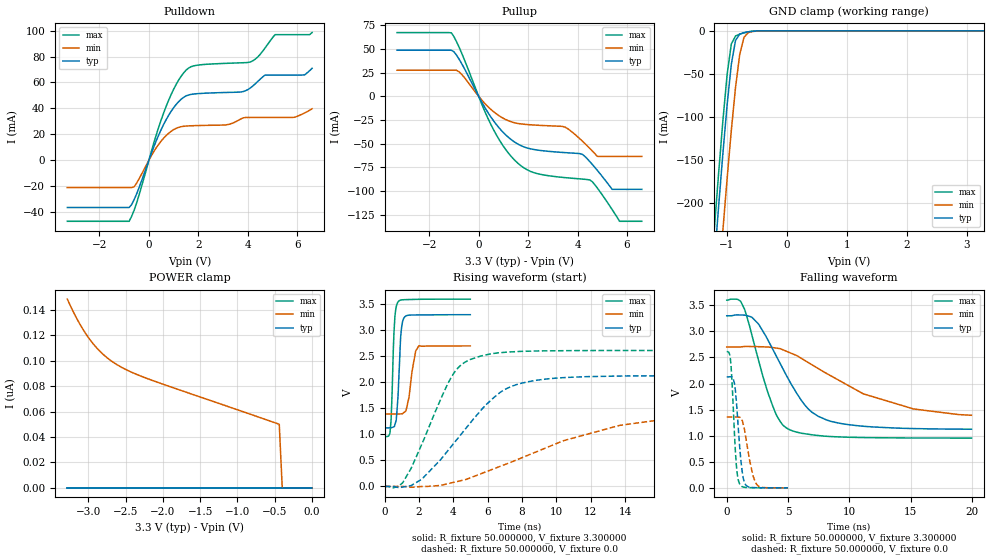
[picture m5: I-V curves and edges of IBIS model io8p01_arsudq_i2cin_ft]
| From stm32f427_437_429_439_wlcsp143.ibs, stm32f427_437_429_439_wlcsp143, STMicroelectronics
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|   Model io8p01_arsudq_i2cin_ft
[Model]  io8p01_arsudq_i2cin_ft
Model_type I/O
Polarity   Non-Inverting
Enable   Active-Low
Vinl =   0.990000V
Vinh =   2.310000V
Vmeas =  1.650000V
Cref =   50.000000pF
Rref =   100.000000M
Vref =   0.0V
C_comp   2.280000pF   2.217100pF   2.355700pF
[Temperature Range]   25.000000   0.125000k   -40.000000
[Pullup Reference]   3.300000V   2.700000V   3.600000V
[Pulldown Reference]   0.0V   0.0V   0.0V
[POWER Clamp Reference]   3.300000V   2.700000V   3.600000V
[GND Clamp Reference]   0.0V   0.0V   0.0V
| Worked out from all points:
|   slope of the pulldown table from 0 to 0.495 V, typ, clamps not added: 20.9 ohm
|   slope of the pullup table from 0 to 0.495 V, typ, clamps not added: 22.6 ohm
|   GND clamp passes 1 mA (typ) near -0.62 V on its own axis
|   rising waveform, R_fixture 50.000000, V_fixture 3.300000: 20-80 % time 192ps typ, 341ps min, 165ps max; typ from 1.12 V to 3.3 V
|   rising waveform, R_fixture 50.000000, V_fixture 0.0: 20-80 % time 3.34ns typ, 6.91ns min, 2.09ns max; typ from 0 V to 2.13 V
|   falling waveform, R_fixture 50.000000, V_fixture 3.300000: 20-80 % time 3.18ns typ, 6.84ns min, 2ns max; typ from 3.3 V to 1.12 V
|   falling waveform, R_fixture 50.000000, V_fixture 0.0: 20-80 % time 434ps typ, 633ps min, 342ps max; typ from 2.13 V to 0 V
[Pulldown]
|Voltage   I(typ)   I(min)   I(max)
-3.3V     -36.46mA   -21.09mA   -47.09mA
-800mV    -36.46mA   -21.09mA   -47.09mA
-600mV    -30.5mA    -20.54mA   -38.69mA
700mV     31.4mA     19.11mA    41.71mA
1.2V      45.15mA    25.37mA    61.75mA
1.6V      50.35mA    26.5mA     71.06mA
3.1V      52.28mA    27.26mA    74.76mA
4.1V      55.7mA     33mA       75.81mA
4.7V      65.72mA    33mA       86.7mA
5.1V      65.72mA    33mA       96.91mA
6.3V      65.88mA    36.51mA    96.91mA
6.6V      70.94mA    39.72mA    98.51mA
[Pullup]
|Voltage   I(typ)   I(min)   I(max)
-3.3V     48.54mA    27.44mA    67.18mA
-1.1V     48.54mA    27.44mA    66.9mA
-700mV    35.13mA    23.47mA    46.35mA
500mV     -22.07mA   -14mA      -30.03mA
1.5V      -49.1mA    -28.3mA    -68.56mA
2.2V      -56.05mA   -30.32mA   -80.35mA
3.5V      -59.53mA   -32.65mA   -85.92mA
4.5V      -69.07mA   -55.12mA   -88.38mA
4.8V      -78.22mA   -63.5mA    -96.83mA
5.4V      -98.3mA    -63.5mA    -119.6mA
5.7V      -98.3mA    -63.5mA    -132mA
6.6V      -98.3mA    -63.5mA    -132mA
[GND_clamp]
|Voltage   I(typ)   I(min)   I(max)
-3.3V     -2.318A    -2.397A    -2.291A
-1.2V     -265.5mA   -356.1mA   -227.2mA
-1.13V    -202.6mA   -292.9mA   -164.1mA
-1.06V    -142.2mA   -231.2mA   -104.1mA
-990mV    -85.98mA   -171.6mA   -50.72mA
-920mV    -38.8mA    -115.5mA   -15.28mA
-850mV    -11.08mA   -65.6mA    -6.001mA
-780mV    -3.782mA   -27.42mA   -3.876mA
-710mV    -2.086mA   -7.69mA    -2.381mA
-640mV    -1.147mA   -2.118mA   -1.22mA
-570mV    -523.9uA   -798.4uA   -476.8uA
3.28V     0A         0A         0A
[POWER_clamp]
|Voltage   I(typ)   I(min)   I(max)
-3.28V    0A         148.5nA    0A
-3.2V     0A         138.6nA    0A
-3.12V    0A         129.7nA    0A
-3.04V    0A         122nA      0A
-2.96V    0A         115.3nA    0A
-2.8V     0A         105.1nA    0A
-2.6V     0A         96.44nA    0A
-2.4V     0A         90.52nA    0A
-2.16V    0A         84.97nA    0A
-440mV    0A         50.04nA    0A
-400mV    0A         0A         0A
0V        0A         0A         0A
[Ramp]
| variable   typ   min   max
dV/dt_r  1.27752/3.33932n   0.79944/6.92058n   1.56720/2.09171n
dV/dt_f  1.30218/3.17757n   0.74058/6.80182n   1.58774/1.99677n
R_load = 50.000000
[Rising Waveform]
R_fixture= 50.000000
V_fixture= 3.300000
V_fixture_min= 2.700000
V_fixture_max= 3.600000
|time   V(typ)   V(min)   V(max)
0s        1.124V     1.392V     954.4mV
300.3ps   1.126V     1.392V     1.023V
370.4ps   1.128V     1.392V     1.3V
500.5ps   1.142V     1.392V     2.655V
590.6ps   1.185V     1.392V     3.262V
760.8ps   1.675V     1.391V     3.538V
930.9ps   2.892V     1.394V     3.581V
1.161ns   3.258V     1.432V     3.588V
1.992ns   3.295V     2.704V     3.596V
4.985ns   3.3V       2.7V       3.599V
[Rising Waveform]
R_fixture= 50.000000
V_fixture= 0.0
V_fixture_min= 0.0
V_fixture_max= 0.0
|time   V(typ)   V(min)   V(max)
0s        358.4uV    205.3uV    679.9uV
1.041ns   -11.38mV   -1.544mV   69.55mV
2.162ns   139.2mV    -2.11mV    815.3mV
3.844ns   754.9mV    64.47mV    2.077V
4.324ns   951.2mV    101.7mV    2.296V
4.965ns   1.212V     162.4mV    2.437V
6.767ns   1.817V     390.4mV    2.571V
8.448ns   2.017V     612.4mV    2.599V
13.69ns   2.12V      1.173V     2.611V
19.94ns   2.129V     1.359V     2.612V
[Falling Waveform]
R_fixture= 50.000000
V_fixture= 3.300000
V_fixture_min= 2.700000
V_fixture_max= 3.600000
|time   V(typ)   V(min)   V(max)
0s        3.3V       2.7V       3.599V
880.9ps   3.315V     2.7V       3.615V
1.441ns   3.311V     2.71V      3.43V
2.563ns   3.148V     2.707V     2.472V
3.724ns   2.669V     2.69V      1.585V
4.965ns   2.11V      2.609V     1.135V
6.647ns   1.513V     2.403V     1.028V
8.488ns   1.275V     2.147V     984mV
15.22ns   1.137V     1.513V     956.6mV
19.94ns   1.124V     1.392V     954.4mV
[Falling Waveform]
R_fixture= 50.000000
V_fixture= 0.0
V_fixture_min= 0.0
V_fixture_max= 0.0
|time   V(typ)   V(min)   V(max)
0s        2.129V     1.359V     2.612V
300.3ps   2.13V      1.359V     2.469V
450.5ps   2.119V     1.358V     1.946V
620.6ps   2.012V     1.358V     1.08V
840.8ps   1.482V     1.361V     295.4mV
1.041ns   824.8mV    1.353V     80.43mV
1.451ns   100.6mV    1.114V     10.56mV
2.132ns   5.392mV    241.2mV    3.409mV
2.422ns   3.511mV    71.5mV     2.73mV
4.985ns   358.4uV    205.3uV    679.9uV
